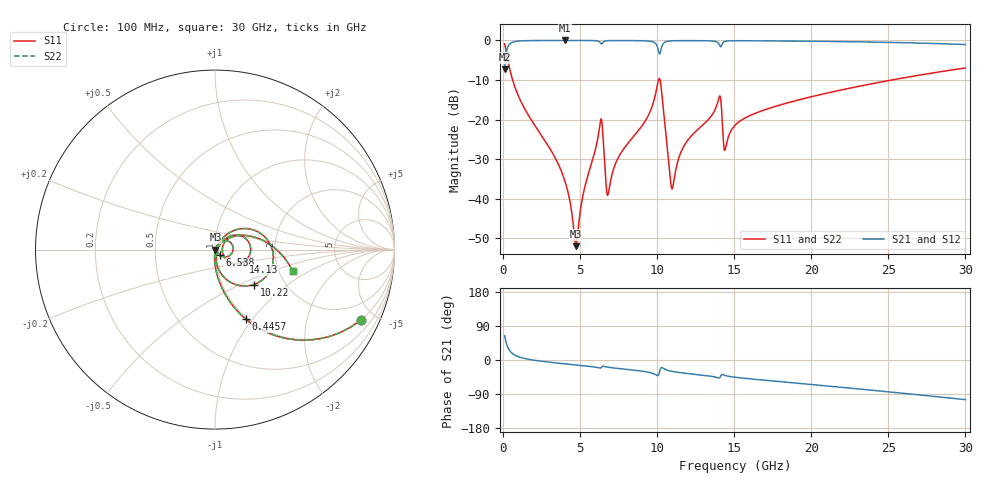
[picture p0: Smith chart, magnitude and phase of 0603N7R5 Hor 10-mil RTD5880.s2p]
# GHz S MA R 50
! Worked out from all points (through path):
!   3201 points, 100 MHz to 30 GHz, reference 50 ohm
!   highest |S21| = -0.02 dB at 3.996 GHz (marker M1); lowest = -7.3 dB at 100 MHz (marker M2)
!   group delay of S21, straight-line fit = 10.3 ps
!   lowest |S11| = -51.9 dB at 4.734 GHz (marker M3), VSWR 1.01, Z = 50.2 - j0.0563 ohm
!   |S11| at or under -10 dB: 621 MHz to 10.08 GHz (9.464 GHz wide, 177 % of centre); 10.19 GHz to 25.22 GHz (15.04 GHz wide, 84.9 % of centre)
!   |S22| runs from -51.9 to -0.9 dB; largest |S21 - S12| = 0
!   S11 on the Smith chart (normalised r, x): 100 MHz: 0.98, -4.16; 445.7 MHz: 0.98, -0.93; 6.538 GHz: 1.06, -0.07; 10.22 GHz: 1.40, -0.60; 14.13 GHz: 1.37, -0.19; 30 GHz: 2.37, -0.71
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0.1  0.903 -25.7  0.4295 64.3  0.4295 64.3  0.903 -25.7
0.4457187  0.4238 -66.1  0.9051 23.8  0.9051 23.8  0.4238 -66.1
1.454844  0.1313 -85.9  0.9901 3.5  0.9901 3.5  0.1313 -85.9
3.996344  0.01714 -92.8  0.9976 -10.0  0.9976 -10.0  0.01714 -92.8
4.7345  0.002527 -12.8  0.9974 -13.0  0.9974 -13.0  0.002527 -12.8
5.089563  0.008782 56.8  0.9971 -14.5  0.9971 -14.5  0.008782 56.8
6.294906  0.08964 30.7  0.9423 -21.3  0.9423 -21.3  0.08964 30.7
6.537844  0.04226 -47.7  0.9635 -16.7  0.9635 -16.7  0.04226 -47.7
6.706031  0.01359 -26.5  0.9865 -18.3  0.9865 -18.3  0.01359 -26.5
6.846188  0.01212 25.9  0.9913 -19.3  0.9913 -19.3  0.01212 25.9
7.509594  0.03406 59.9  0.9948 -22.5  0.9948 -22.5  0.03406 59.9
9.369  0.1074 52.2  0.9827 -31.7  0.9827 -31.7  0.1074 52.2
10.06978  0.3084 5.9  0.7616 -40.4  0.7616 -40.4  0.3084 5.9
10.21928  0.2915 -42.0  0.7206 -22.2  0.7206 -22.2  0.2915 -42.0
10.97612  0.0134 -11.8  0.9871 -30.1  0.9871 -30.1  0.0134 -11.8
11.84509  0.05025 47.6  0.9922 -35.1  0.9922 -35.1  0.05025 47.6
14.13431  0.1741 -22.9  0.8332 -41.5  0.8332 -41.5  0.1741 -22.9
14.42397  0.04273 13.3  0.9743 -41.0  0.9743 -41.0  0.04273 13.3
15.05  0.08479 39.7  0.9892 -45.5  0.9892 -45.5  0.08479 39.7
20.03956  0.1951 23.7  0.9752 -64.8  0.9752 -64.8  0.1951 23.7
25.01978  0.311 4.8  0.9438 -84.0  0.9438 -84.0  0.311 4.8
30  0.4492 -15.5  0.8858 -104.6  0.8858 -104.6  0.4492 -15.5
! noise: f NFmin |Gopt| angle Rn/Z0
0.1  0.0003394  0.9298  0.5968  0.001074
3.417  0.003821  0.8003  9.447  0.003939
6.743  0.01307  0.8802  18.49  0.02302
10.06  0.07426  0.9673  27.45  0.4855
13.39  0.01561  0.8111  36.18  0.01558
16.7  0.01355  0.7416  44.64  0.009032
20.03  0.01524  0.7298  52.92  0.009057
23.35  0.01742  0.7281  60.98  0.009547
26.67  0.01982  0.7303  68.85  0.01008
30  0.02246  0.7352  76.5  0.0106
